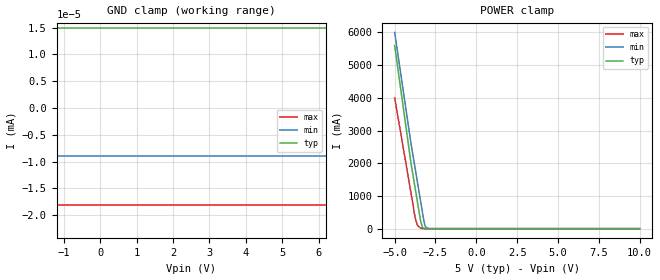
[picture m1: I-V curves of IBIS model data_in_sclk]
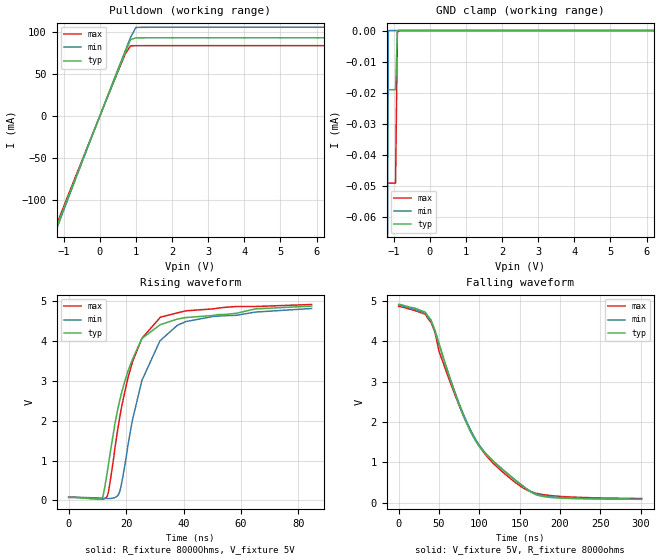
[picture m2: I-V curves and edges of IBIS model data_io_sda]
[IBIS Ver]   4.0
[File name]   fs23_i2c.ibs
[File Rev]   1.1
[Date]   MARCH 2025
[Source]   NXP semiconductors
[Notes]   IBIS model for the fs23 includes the model of I2C pins
|   .SCLK. SDA
[Disclaimer]   This information is for modeling purposes only
|   and is not guaranteed.The simulation model is not able to
|   reproduce identically the quality structure
|   and behavior of the final product.
[Copyright]   Copyright 2021 NXP Semiconductors: All Rights Reserved. This
|   simulation model or derivative thereof is the proprietary
|   information of NXP Semiconductors. is confidential in nature
|   and may not be reproduced in any way
|   (physically or electronically)
|   without the express permission from NXP Semiconductors.
[Component]   fs23_i2c
[Manufacturer]   NXP semiconductors
[Package]
|   typ   min   max
R_pkg   0.083216   0.072192   0.098491
L_pkg   1.928e-9   1.494e-9   2.406e-9
C_pkg   2.869e-13   2.631e-13   3.056e-13
[Pin]   Signal_name   model_name   R_pin   L_pin   C_pin
28   SDA   data_io_sda   0.072192   1.494e-9   2.631e-13
27   SCK   data_in_sclk   0.075468   1.744e-9   2.79e-13
| end pin list
| Models and submodels in the file (2): data_in_sclk (Input), data_io_sda (I/O_open_drain)
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|   Model data_in_sclk
[Model]   data_in_sclk
Model_type   Input
Polarity   Non-Inverting
|   typ   min   max
C_comp   85.91f   82.40f   97.09f
| Where typ is typical value of c_comp (no PVT)
|   min is the minimum value of c_comp under PVT
|   max is the maximum value of c_comp under PVT
Vinh  =   2.50
Vinl  =   2.11
| Hysteresis
|   |   Rising Edge   Falling Edge
|   |   Switching Region   oo   o   Switching Region
|   |   |  o   oo  ooooooooo   |
|   |   V o   o   |
| Vinh  - - - - - - - - - - x   o   |
|   |   o   o  |
|   |   o   o |
|   |   o   oV
| Vinl  - - - - - - -  o - - - - - - - - - - - - - - - - - x
|   |   o   o
|   |   o   o
|   |oooooo-----------------------------------------------------oooooooo
|   typ   min   max
[Temperature Range]   27   -40   175
|   typ   min   max
[Voltage Range]   5V   4.91V   5.2V
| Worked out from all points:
|   POWER clamp passes 1 mA (typ) near -3.10 V on its own axis
[GND Clamp]
|Voltage   I(typ)   I(min)  I(max)
-5V       -6.4A      -6.7A      -5.7A
-1.6V     -200mA     -400mA     -10mA
-1.5V     -100mA     -250mA     -18nA
-1.4V     -50mA      -150mA     -18nA
-1.3V     15nA       -50mA      -18nA
-1.2V     15nA       -9nA       -18nA
10V       15nA       -9nA       -18nA
[POWER Clamp]
|Voltage   I(typ)   I(min)  I(max)
-5V       5.6A       6A         4A
-4V       2A         2.6A       1.09A
-3.8V     1.4A       2A         480mA
-3.7V     1.1A       1.7A       250mA
-3.6V     800mA      1.4A       100mA
-3.4V     200mA      800mA      15mA
-3.3V     50mA       500mA      5mA
-3.15V    5mA        100mA      2.2nA
-3.1V     1mA        50mA       2.2nA
-2.8V     1.4nA      1.2nA      2.2nA
10V       1.4nA      1.2nA      2.2nA
|   Model data_io_sda
[Model]   data_io_sda
Model_type   I/O_open_drain
Polarity   Non-Inverting
|   typ   min   max
C_comp   1.78p   1.17p   2.35p
| Where typ is typical value of c_comp (no PVT)
|   min is the minimum value of c_comp under PVT
|   max is the maximum value of c_comp under PVT
Vinh  =   2.505
Vinl  =   2.114
[Temperature Range]   27   -40   175
|   typ   min   max
[Voltage Range]   5V   4.91V   5.2V
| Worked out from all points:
|   slope of the pulldown table from 0 to 0.75 V, typ, clamps not added: 9.33 ohm
|   GND clamp passes 1 mA (typ) near -1.31 V on its own axis
|   rising waveform, R_fixture 8000Ohms, V_fixture 5V: 20-80 % time 10.4ns typ, 11ns min, 9.22ns max; typ from 0.074 V to 4.87 V
|   falling waveform, V_fixture 5V, R_fixture 8000ohms: 20-80 % time 65.8ns typ, 66.5ns min, 65.2ns max; typ from 4.91 V to 0.085 V
[GND Clamp]
|Voltage   I(typ)   I(min)   I(max)
-5V       -6.37A     -6.706A    -5.62A
-1.55V    -154mA     -300mA     -5mA
-1.5V     -100mA     -256mA     -49uA
-1.35V    -5mA       -89mA      -49uA
-1.3V     -19uA      -40mA      -49uA
-1.2V     -19uA      -163uA     -49uA
-1.15V    -19uA      -19nA      -49uA
-950mV    -19uA      85pA       -49uA
-900mV    -83pA      85pA       -670nA
-850mV    -83pA      85pA       366pA
10V       -83pA      85pA       366pA
[Pulldown]
|   typ   min   max
-5V       -529.9mA   -548.8mA   -515.9mA
-1.4V     -153.9mA   -157.1mA   -150.9mA
-1.25V    -137.2mA   -140.1mA   -134.6mA
-1.1V     -120.6mA   -123.1mA   -118.3mA
-200mV    -21.74mA   -22.2mA    -21.3mA
700mV     75.1mA     77.02mA    73.37mA
850mV     90.66mA    93.35mA    83.23mA
1V        92.67mA    105.1mA    83.37mA
10V       92.74mA    105.3mA    83.42mA
[Rising Waveform]
R_fixture = 8000Ohms
V_fixture = 5V
|time   V(typ)   V(min)   V(max)
0s        74.1mV     82.3mV     81.4mV
11.9ns    94.3mV     57.1mV     35.9mV
13.8ns    877mV      49.15mV    199mV
17.3ns    2.351V     144mV      1.874V
18.8ns    2.789V     557mV      2.461V
20.6ns    3.232V     1.366V     3.061V
25.5ns    4.059V     3.007V     4.062V
31.9ns    4.405V     4.007V     4.59V
40.8ns    4.583V     4.482V     4.751V
84.6ns    4.87V      4.81V      4.91V
[Falling Waveform]
V_fixture = 5V
R_fixture = 8000ohms
|time   V(typ)   V(min)   V(max)
0s        4.91V      4.89V      4.86V
33ns      4.72V      4.69V      4.67V
40ns      4.53V      4.5V       4.47V
60ns      3.295V     3.305V     3.193V
75ns      2.417V     2.457V     2.407V
90ns      1.725V     1.769V     1.744V
109ns     1.182V     1.199V     1.155V
140ns     633.4mV    637.4mV    573.8mV
180ns     151.1mV    171.4mV    197.9mV
301ns     84.53mV    90.05mV    104.7mV
[Ramp]
R_load = 8000ohms
|   typ   min   max
dV/dt_r   0.239/1e-9   0.236/1e-9   0.241/1e-9
dV/dt_f   7.854/1e-3   4.681/1e-3   11.02/1e-3
|  end [Model]   data_io_sda
